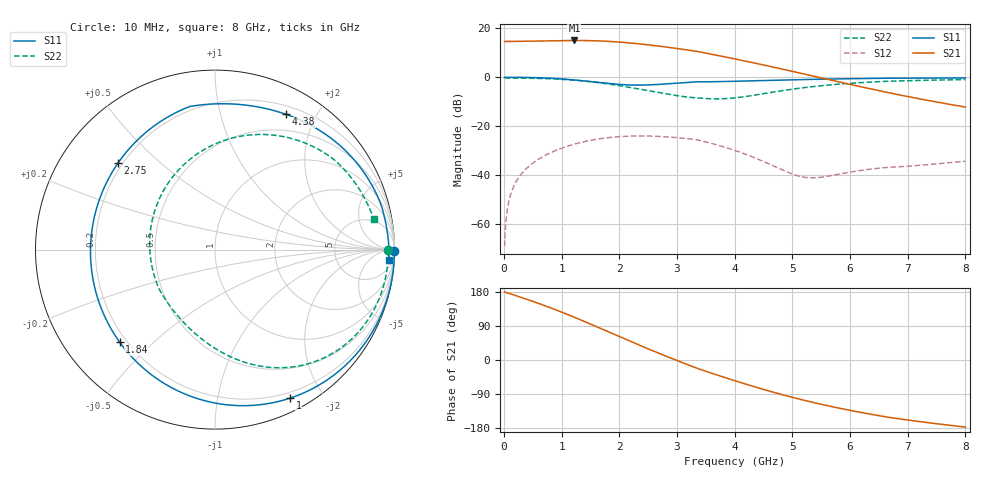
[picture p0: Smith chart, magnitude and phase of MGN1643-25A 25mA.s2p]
! Port[1] = GATE
! Port[2] = DRAIN
! [Type]  S-parameter s2p file touchstone ver. 1.0
! [Object]  MGN1643-25A
! [Bias]  25 mA
! [Version]  1.0
! [Date]  Tue May 19 13:03:48 2026
! [Source]  This file was created in JSC "ICC Milandr".
! [Disclaimer] Property of JSC "ICC Milandr". Unauthorized reproduction and/or distribution is strictly prohibited.
!  The file and the data are provided "AS IS" and with all faults and disclaim all warranties, express and implied, including
!  without limitation any implied warranties of merchantability, fitness for a particular purpose.
!  JSC "ICC Milandr" assumes no liability for:
!  1) the accuracy of the data provided;
!  2) the proper functioning of this data;
!  3) infringement of patents, copyrights or intellectual property rights resulting from the use of this data.
!  JSC "ICC Milandr" reserves the right to make changes to the products and the data without prior notice.
!  Please, be aware that your receipt and use of the file provided shall serve as acceptance of these terms and conditions.
!  If you do not accept these terms, you should return or destroy this file and any other accompanying information immediately.
# Hz S MA R 12.5
! freq  S11mag  S11ang  S21mag  S21ang  S12mag  S12ang  S22mag  S22ang
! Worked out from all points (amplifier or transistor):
!   800 points, 10 MHz to 8 GHz, reference 12.5 ohm
!   highest |S21| = 15.1 dB at 1.22 GHz (marker M1)
!   |S21| within 3 dB of that: start of sweep to 2.908 GHz
!   unconditionally stable (mu >= 1): 3.545 GHz to end of sweep
!   at 1.34 GHz: K = 0.37, MSG = 20.8 dB, |S12| = -26.6 dB
!   at 4.01 GHz: K = 1.59, MAG = 14.2 dB, |S12| = -30.0 dB
!   at 8 GHz: K = 1.10, MAG = 9.1 dB, |S12| = -34.3 dB
!   S11 on the Smith chart (normalised r, x): 10 MHz: open; 1 GHz: 0.14, -1.62; 1.84 GHz: 0.17, -0.39; 2.75 GHz: 0.18, +0.37; 4.38 GHz: 0.30, +1.62; 8 GHz: 14, -28
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1e7  0.9999 -0.6  5.412 179.5  0.0003527 83.2  0.9659 -0.3
1e8  0.9999 -5.8  5.412 175.1  0.003496 84.9  0.9658 -3.2
2.5e8  0.998 -14.5  5.434 167.7  0.008763 78.5  0.9639 -7.9
6.4e8  0.9766 -38.4  5.544 147.1  0.0227 59.9  0.9471 -20.7
1e9  0.9276 -63.1  5.647 126.3  0.03559 40.9  0.9095 -33.3
1.22e9  0.8832 -80.0  5.671 112.7  0.04306 28.4  0.8735 -41.4
1.35e9  0.8531 -90.6  5.66 104.5  0.04715 20.8  0.8474 -46.3
1.59e9  0.7948 -111.9  5.581 88.9  0.05375 6.4  0.7904 -55.5
1.84e9  0.7402 -135.9  5.409 72.3  0.05892 -8.9  0.7219 -65.3
2.26e9  0.6941 -178.0  4.942 44.7  0.06305 -34.6  0.5992 -82.4
2.47e9  0.6979 162.0  4.653 31.2  0.06306 -47.2  0.5407 -91.6
2.68e9  0.716 143.9  4.349 18.1  0.06192 -59.5  0.4874 -101.8
2.75e9  0.7242 138.3  4.246 13.7  0.06132 -63.5  0.4711 -105.5
3.03e9  0.7633 118.2  3.838 -3.2  0.05801 -79.4  0.4159 -122.3
3.35e9  0.8096 99.5  3.384 -22.0  0.05267 -97.2  0.3792 -146.3
3.66e9  0.8145 86.1  2.869 -37.9  0.04253 -108.8  0.3621 -171.0
4.01e9  0.8297 73.5  2.37 -55.1  0.03176 -119.4  0.3806 158.9
4.38e9  0.8513 62.3  1.919 -72.3  0.02177 -126.0  0.4388 130.2
4.84e9  0.8799 50.3  1.459 -92.1  0.01253 -121.1  0.5372 101.7
5.34e9  0.9079 39.1  1.073 -111.3  0.008798 -90.5  0.6428 78.3
6.67e9  0.9585 15.1  0.4841 -151.3  0.01445 -64.1  0.8321 36.9
8e9  0.972 -3.3  0.246 -176.9  0.01919 -85.7  0.9003 10.9
